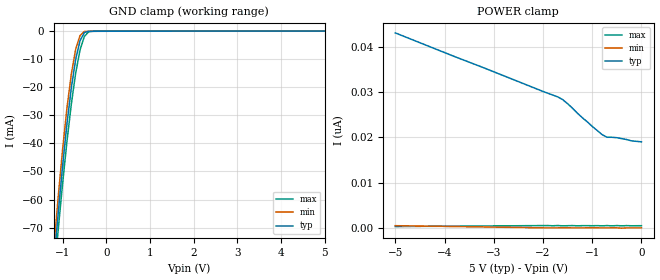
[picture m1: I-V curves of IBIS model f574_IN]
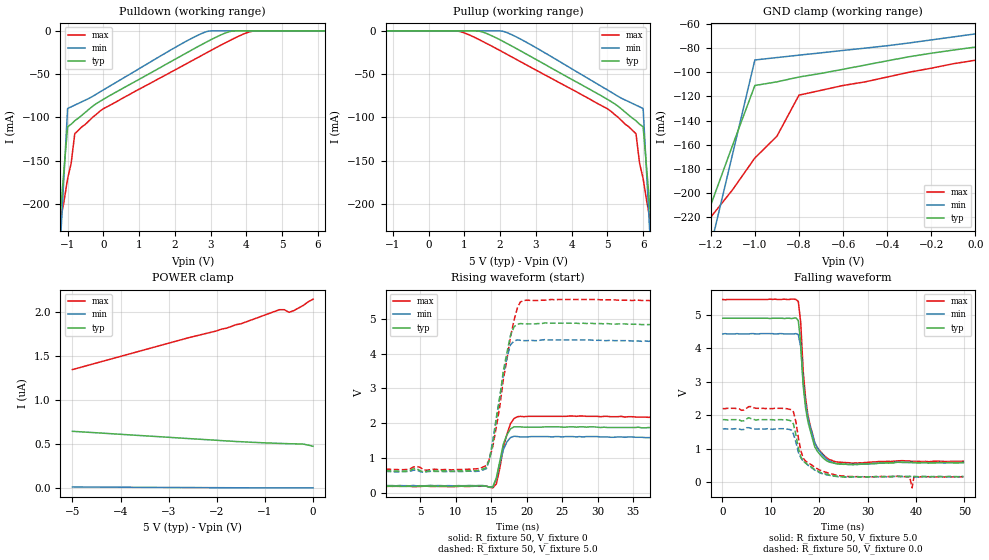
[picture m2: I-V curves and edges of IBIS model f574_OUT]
| TEXAS INSTRUMENTS INCORPORATED
| Standard Linear and Logic Group
| IBIS Model of SN74F574
| OCTAL EDGE-TRIGGERED D-TYPE FLIP-FLOPS WITH 3-STATE OUTPUTS
| SOP 20-pin (NS), SSOP 20-pin (DB)
[IBIS Ver]   3.0
[Comment Char]  |_char
[File Name]   f574.ibs
[File Rev]   2.0 I_die
[Date]   Aug 03, 2000
[Source]   File originated at Texas Instruments, Inc.
[Notes]   The following is a sample IBIS file for the F574
|   - All test data contained in this file are derived from
|   actual measurements.
|   - File created by Nobuhisa Ohtsubo, SLL Product Engineering.
[Disclaimer] Property of Texas Instruments Incorporated.  Unauthorized
   reproduction and/or distribution is strictly prohibited.
   This product is protected under copyright law.
   Created 2000, (C) Copyright 2000, Texas Instruments Inc.,
   All Rights Reserved.
   UNLESS THERE IS A SIGNED, WRITTEN AGREEMENT TO THE
   CONTRARY, TEXAS INSTRUMENTS () IS PROVIDING THE IBIS
   MODELS  AND WITHOUT ANY WARRANTY, EXPRESSED OR
   IMPLIED.  TI assumes no liability for:
   1) the accuracy of the IBIS models provided to your
   company;
   2) the proper functioning of these IBIS Models in your
   design or for any resulting applications; or
   3) infringement of patents, copyrights or intellectual
   property rights resulting from your use of these IBIS
   models.
   TI provides IBIS Models as a service to our customers.
   You and your company shall not distribute, sell or give
   these models to anyone else without prior written
   permission from TI.
   TI reserves the right to make changes to our products or
   to discontinue any semiconductor product or service
   without notice, and advises our customers to obtain the
   latest version of relevant information to verify, before
   placing orders, that the information being relied on is
   current.
   Please be aware that your receipt and use of the IBIS
   information provided shall serve as acceptance of these
   terms and conditions.  If you do not accept these terms,
   you should return or destroy the IBIS models and any
   other accompanying information immediately.
|   Component F574_NS
[Component]   f574_NS
[Manufacturer]  Texas Instruments, Inc.
[Package]
|   typ   min   max
R_pkg   0.044   0.029   0.058
L_pkg   3.666nH   2.317nH   5.115nH
C_pkg   0.548pF   0.316pF   0.725pF
[Pin]   signal_name   model_name   R_pin   L_pin   C_pin
1   OE_NOT   f574_IN   0.058   5.115nH   0.725pF
2   1D   f574_IN   0.053   4.591nH   0.724pF
3   2D   f574_IN   0.049   3.754nH   0.572pF
4   3D   f574_IN   0.029   2.549nH   0.388pF
5   4D   f574_IN   0.031   2.317nH   0.316pF
6   5D   f574_IN   0.031   2.317nH   0.316pF
7   6D   f574_IN   0.029   2.556nH   0.399pF
8   7D   f574_IN   0.049   3.754nH   0.579pF
9   8D   f574_IN   0.053   4.591nH   0.724pF
10   GND   GND   0.058   5.115nH   0.725pF
11   CLK   f574_IN   0.058   5.115nH   0.725pF
12   8Q   f574_OUT   0.053   4.591nH   0.724pF
13   7Q   f574_OUT   0.049   3.754nH   0.579pF
14   6Q   f574_OUT   0.029   2.557nH   0.399pF
15   5Q   f574_OUT   0.031   2.317nH   0.316pF
16   4Q   f574_OUT   0.031   2.317nH   0.316pF
17   3Q   f574_OUT   0.029   2.557nH   0.399pF
18   2Q   f574_OUT   0.049   3.754nH   0.579pF
19   1Q   f574_OUT   0.053   4.591nH   0.724pF
20   VCC   POWER   0.058   5.115nH   0.725pF
|   Component F574_DB
[Component]   f574_DB
[Manufacturer]  Texas Instruments, Inc.
[Package]
|   typ   min   max
R_pkg   0.040   0.035   0.051
L_pkg   3.495nH   3.035nH   4.314nH
C_pkg   0.420pF   0.346pF   0.502pF
[Pin]   signal_name   model_name   R_pin   L_pin   C_pin
1   OE_NOT   f574_IN   0.049   4.310nH   0.502pF
2   1D   f574_IN   0.048   3.903nH   0.487pF
3   2D   f574_IN   0.035   3.189nH   0.396pF
4   3D   f574_IN   0.035   3.036nH   0.347pF
5   4D   f574_IN   0.035   3.035nH   0.367pF
6   5D   f574_IN   0.035   3.035nH   0.367pF
7   6D   f574_IN   0.035   3.036nH   0.347pF
8   7D   f574_IN   0.035   3.189nH   0.397pF
9   8D   f574_IN   0.047   3.899nH   0.488pF
10   GND   GND   0.051   4.314nH   0.500pF
11   CLK   f574_IN   0.051   4.314nH   0.500pF
12   8Q   f574_OUT   0.047   3.899nH   0.488pF
13   7Q   f574_OUT   0.035   3.189nH   0.397pF
14   6Q   f574_OUT   0.035   3.036nH   0.346pF
15   5Q   f574_OUT   0.035   3.035nH   0.367pF
16   4Q   f574_OUT   0.035   3.035nH   0.367pF
17   3Q   f574_OUT   0.035   3.036nH   0.346pF
18   2Q   f574_OUT   0.035   3.189nH   0.397pF
19   1Q   f574_OUT   0.047   3.899nH   0.488pF
20   VCC   POWER   0.051   4.314nH   0.502pF
| Models and submodels in the file (2): f574_IN (Input), f574_OUT (3-state)
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|   Model F574_IN
[Model]   f574_IN
Model_type  Input
Polarity   Inverting
Vinl = 0.8
Vinh = 2.0
| variable   typ   min   max
C_comp   1.33pf   1.00pf   1.66pf
[Temperature Range]   25   0   70
[Voltage Range]   5.0   4.75   5.25
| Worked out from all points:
|   GND clamp passes 1 mA (typ) near -0.52 V on its own axis
[GND Clamp]
|   Voltage   I(typ)   I(min)   I(max)
-5V       -1.02A     -1.07A     -940mA
-1.2V     -82.9mA    -77.6mA    -88.1mA
-1.1V     -64.9mA    -59.1mA    -70.8mA
-1V       -48.2mA    -42.3mA    -54.5mA
-900mV    -33.1mA    -27.5mA    -39.4mA
-800mV    -20.3mA    -15.4mA    -26.1mA
-700mV    -10.1mA    -6.49mA    -15mA
-600mV    -3.44mA    -1.57mA    -6.7mA
-500mV    -512uA     -145uA     -1.86mA
-400mV    -83.7uA    -69.8uA    -240uA
-300mV    -64.3uA    -65.2uA    -68.9uA
5V        19nA       36.1pA     510pA
[POWER Clamp]
|   Voltage   I(typ)   I(min)   I(max)
-5V       43nA       516pA      326pA
-2V       30.1nA     40.9pA     537pA
-1.7V     28.9nA     37pA       555pA
-1.6V     28.3nA     48pA       475pA
-1.5V     27.4nA     48.4pA     510pA
-1.2V     24.3nA     32.4pA     520pA
-800mV    20.6nA     25.5pA     473pA
-700mV    20nA       28.7pA     538pA
-600mV    20nA       41.2pA     469pA
-500mV    19.9nA     43.9pA     547pA
-200mV    19.2nA     24.6pA     489pA
0V        19nA       36.1pA     510pA
|   Model F574_OUT
[Model]   f574_OUT
Model_type  3-state
Polarity   Non-Inverting
Enable   Active-Low
Vmeas = 1.5v
Cref = 0pf
| variable   typ   min   max
C_comp   5.8pf   4.35pf   7.25pf
[Temperature Range]   25   0   70
[Voltage Range]   5.0   4.5   5.5
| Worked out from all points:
|   slope of the pulldown table from 0 to 0.75 V, typ, clamps not added: 43 ohm
|   rising waveform, R_fixture 50, V_fixture 0: 20-80 % time 1.15ns typ, 1.06ns min, 1.3ns max; typ from 0.197 V to 1.88 V
|   falling waveform, R_fixture 50, V_fixture 5.0: 20-80 % time 2.1ns typ, 2.38ns min, 2.05ns max; typ from 4.9 V to 0.591 V
|   rising waveform, R_fixture 50, V_fixture 5.0: 20-80 % time 1.93ns typ, 1.83ns min, 2.31ns max; typ from 0.635 V to 4.85 V
|   falling waveform, R_fixture 50, V_fixture 0.0: 20-80 % time 2.69ns typ, 3.25ns min, 2.6ns max; typ from 1.87 V to 0.179 V
[Pulldown]
|   Voltage   I(typ)   I(min)   I(max)
-5V       -2.07A     -3.16A     -1.12A
-1.3V     -259mA     -320mA     -244mA
-1.2V     -210mA     -244mA     -220mA
-1.1V     -160mA     -167mA     -197mA
-1V       -111mA     -89.9mA    -171mA
-900mV    -108mA     -87.9mA    -153mA
-800mV    -104mA     -85.9mA    -119mA
-600mV    -97.6mA    -82mA      -111mA
2.8V      -14.8mA    -2.17mA    -27.3mA
3.5V      -1.22mA    7.6nA      -12mA
4.2V      483nA      6.11nA     -217uA
10V       649nA      17nA       1.35uA
[Pullup]
|   Voltage   II(typ)   I(min)   I(max)
-5V       649nA      17nA       1.35uA
800mV     483nA      6.11nA     -217uA
1.5V      -1.22mA    7.6nA      -12mA
2.2V      -14.8mA    -2.17mA    -27.3mA
5.6V      -97.6mA    -82mA      -111mA
5.8V      -104mA     -85.9mA    -119mA
5.9V      -108mA     -87.9mA    -153mA
6V        -111mA     -89.9mA    -171mA
6.1V      -160mA     -167mA     -197mA
6.2V      -210mA     -244mA     -220mA
6.3V      -259mA     -320mA     -244mA
10V       -2.07A     -3.16A     -1.12A
[GND Clamp]
|   Voltage   I(typ)   I(min)   I(max)
-5V       -2.07A     -3.16A     -1.12A
-1.3V     -259mA     -320mA     -244mA
-1.2V     -210mA     -244mA     -220mA
-1.1V     -160mA     -167mA     -197mA
-1V       -111mA     -89.9mA    -171mA
-900mV    -108mA     -87.9mA    -153mA
-800mV    -104mA     -85.9mA    -119mA
-300mV    -87.2mA    -75.8mA    -100mA
0V        -79.2mA    -68.3mA    -90.1mA
[POWER Clamp]
|   Voltage   I(typ)   I(min)   I(max)
-5V       649nA      17nA       1.35uA
-2.6V     567nA      10.5nA     1.71uA
-1.8V     540nA      8.36nA     1.82uA
-1.6V     533nA      7.92nA     1.86uA
-1.5V     531nA      7.83nA     1.87uA
-700mV    512nA      7.05nA     2.03uA
-600mV    510nA      6.98nA     2.03uA
-500mV    508nA      7.01nA     2uA
-400mV    507nA      6.91nA     2.02uA
-200mV    504nA      6.98nA     2.08uA
-100mV    492nA      7nA        2.12uA
0V        479nA      7.08nA     2.15uA
[Ramp]
| variable   typ   min   max
dV/dt_r   1.032/1.106n   0.852/1.028n   1.224/1.273n
dV/dt_f   2.652/2.092n   2.364/2.401n   2.970/2.028n
R_load = 50
[Rising Waveform]
R_fixture = 50
V_fixture = 0
|   Time   V(typ)   V(min)   V(max)
97.7ps    197mV      216mV      190mV
15.2ns    174mV      181mV      150mV
15.7ns    432mV      400mV      262mV
16.2ns    920mV      857mV      720mV
16.7ns    1.41V      1.25V      1.31V
17.2ns    1.67V      1.47V      1.69V
17.7ns    1.84V      1.59V      1.99V
18.2ns    1.9V       1.63V      2.14V
18.7ns    1.9V       1.62V      2.19V
49.8ns    1.88V      1.6V       2.18V
[Falling Waveform]
R_fixture = 50
V_fixture = 5.0
V_fixture_min = 4.5
V_fixture_max = 5.5
|   Time   V(typ)   V(min)   V(max)
97.7ps    4.9V       4.43V      5.46V
15.7ns    4.83V      4.41V      5.4V
16.2ns    4.15V      4.04V      4.77V
16.7ns    2.89V      3V         3.33V
17.2ns    2.22V      2.36V      2.51V
17.7ns    1.8V       1.92V      1.99V
19.1ns    1.06V      1.18V      1.18V
22.1ns    604mV      642mV      678mV
27ns      526mV      532mV      568mV
49.8ns    591mV      590mV      630mV
[Rising Waveform]
R_fixture = 50
V_fixture = 5.0
V_fixture_min = 4.5
V_fixture_max = 5.5
|   Time   V(typ)   V(min)   V(max)
97.7ps    635mV      619mV      686mV
14.3ns    733mV      699mV      791mV
15.2ns    1.41V      1.5V       1.33V
16.2ns    2.75V      2.78V      2.5V
16.7ns    3.52V      3.42V      3.27V
17.2ns    4.03V      3.88V      3.84V
17.7ns    4.52V      4.25V      4.48V
18.2ns    4.77V      4.36V      4.96V
19.1ns    4.86V      4.38V      5.48V
49.8ns    4.85V      4.37V      5.56V
[Falling Waveform]
R_fixture = 50
V_fixture = 0.0
|   Time   V(typ)   V(min)   V(max)
97.7ps    1.87V      1.59V      2.2V
14.3ns    1.83V      1.56V      2.17V
15.2ns    1.42V      1.2V       1.81V
15.7ns    1.02V      900mV      1.34V
16.7ns    636mV      634mV      719mV
22.1ns    219mV      210mV      263mV
38.7ns    176mV      175mV      164mV
39.2ns    174mV      170mV      -166mV
39.6ns    170mV      162mV      172mV
49.8ns    179mV      169mV      164mV
